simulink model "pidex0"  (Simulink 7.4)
settings: Solver=ode45  StartTime=0.0  StopTime=100  MaxStep=1e-3  RelTol=1e-3
libraries: simulink x2

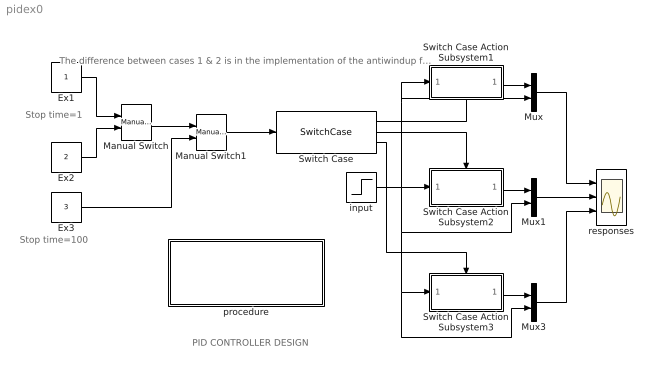
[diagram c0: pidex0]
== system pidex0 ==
  note: PID CONTROLLER DESIGN
  note: The difference between cases 1 & 2 is in the implementation of the antiwindup feature
  note: Stop time=1
  note: Stop time=100
  Ex1 : Constant  OutDataType=sfix(16)  OutScaling=2^0
  Ex2 : Constant  Value=2  OutDataType=sfix(16)  OutScaling=2^0
  Ex3 : Constant  Value=3  OutDataType=sfix(16)  OutScaling=2^0
  Manual Switch : simulink/Signal Routing/Manual Switch  SystemSampleTime=-1  sw=0  action=0  varsize=off
  Manual Switch1 : simulink/Signal Routing/Manual Switch  SystemSampleTime=-1  sw=0  action=0  varsize=off
  Mux : Mux  Inputs=2
  Mux1 : Mux  Inputs=2
  Mux3 : Mux  Inputs=2
  Switch Case : SwitchCase  CaseConditions={1,2,3}  ShowDefaultCase=off
  Switch Case Action Subsystem1 : Subsystem  TreatAsAtomicUnit=on
  Switch Case Action Subsystem2 : Subsystem  TreatAsAtomicUnit=on
  Switch Case Action Subsystem3 : Subsystem  TreatAsAtomicUnit=on
  input : Step  Time=.05  SampleTime=0
  procedure : Subsystem
  responses : Scope  NumInputPorts=3
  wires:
  Ex1/1 -> Manual Switch/1
  Ex2/1 -> Manual Switch/2
  Switch Case/2 -> Switch Case Action Subsystem2/Action
  Switch Case/1 -> Switch Case Action Subsystem1/Action
  input/1 -> Switch Case Action Subsystem2/1(In1), Mux1/2, Mux3/2, Switch Case Action Subsystem3/1(In1), Switch Case Action Subsystem1/1(In1), Mux/2
  Switch Case Action Subsystem1/1(Out1) -> Mux/1
  Switch Case Action Subsystem2/1(Out1) -> Mux1/1
  Mux1/1 -> responses/2
  Switch Case Action Subsystem3/1(Out1) -> Mux3/1
  Mux/1 -> responses/1
  Mux3/1 -> responses/3
  Switch Case/3 -> Switch Case Action Subsystem3/Action
  Manual Switch/1 -> Manual Switch1/1
  Manual Switch1/1 -> Switch Case/1
  Ex3/1 -> Manual Switch1/2

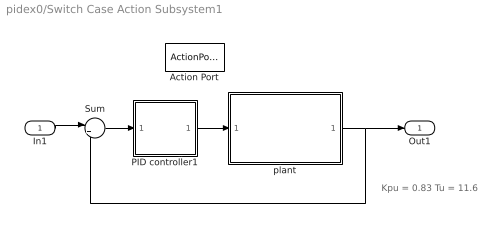
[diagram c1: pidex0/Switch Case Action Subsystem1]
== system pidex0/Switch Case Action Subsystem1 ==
  note: Kpu = 0.83 Tu = 11.6
  In1 : Inport  OutDataType=sfix(16)  OutScaling=2^0
  Action Port : ActionPort  ActionType=case
  PID controller1 : Subsystem  mask{Kp=5.1, Ki=53.7, Kd=0.11, sat=1.8}
      mask prompts: Kp "Proportional gain (Kp)"; Ki "Integral gain (Ki)"; Kd "Derivative gain (Kd)"; sat "Saturation limit [pu]"
      mask help: Proportional-Integral Speed Controller
  Sum : Sum  Inputs=|+-  OutDataType=sfix(16)  OutScaling=2^0
  plant : Subsystem  mask{Ka=1, Ta=0.25, Td=0.05}
      mask prompts: Ka "Gain"; Ta "Time constant [s]"; Td "Time delay [s]"
  Out1 : Outport
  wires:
  In1/1 -> Sum/1
  PID controller1/1(c) -> plant/1(In1)
  Sum/1 -> PID controller1/1(er)
  plant/1(Out1) -> Out1/1, Sum/2

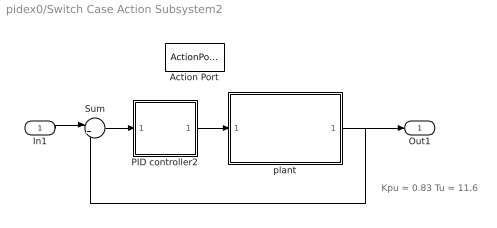
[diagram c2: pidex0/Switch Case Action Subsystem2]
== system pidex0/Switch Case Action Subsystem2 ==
  note: Kpu = 0.83 Tu = 11.6
  In1 : Inport  OutDataType=sfix(16)  OutScaling=2^0
  Action Port : ActionPort  ActionType=case
  PID controller2 : Subsystem  mask{Kp=5.1, Ki=53.7, Kd=0.11, sat=1.8}
      mask prompts: Kp "Proportional gain (Kp)"; Ki "Integral gain (Ki)"; Kd "Derivative gain (Kd)"; sat "Saturation limit [pu]"
      mask help: Proportional-Integral Speed Controller
  Sum : Sum  Inputs=|+-  OutDataType=sfix(16)  OutScaling=2^0
  plant : Subsystem  mask{Ka=1, Ta=0.25, Td=0.05}
      mask prompts: Ka "Gain"; Ta "Time constant [s]"; Td "Time delay [s]"
  Out1 : Outport
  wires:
  PID controller2/1(c) -> plant/1(In1)
  Sum/1 -> PID controller2/1(er)
  plant/1(Out1) -> Out1/1, Sum/2
  In1/1 -> Sum/1

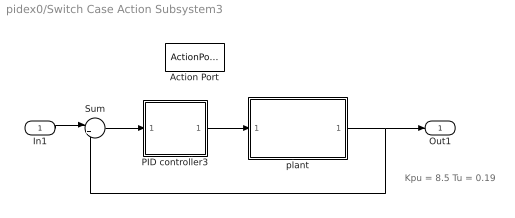
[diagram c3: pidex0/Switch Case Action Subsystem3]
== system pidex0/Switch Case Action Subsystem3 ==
  note: Kpu = 8.5 Tu = 0.19
  In1 : Inport  OutDataType=sfix(16)  OutScaling=2^0
  Action Port : ActionPort  ActionType=case
  PID controller3 : Subsystem  mask{Kp=0.5, Ki=0.09, Kd=0.77, sat=inf}
      mask prompts: Kp "Proportional gain (Kp)"; Ki "Integral gain (Ki)"; Kd "Derivative gain (Kd)"; sat "Saturation limit [pu]"
      mask help: Proportional-Integral Speed Controller
  Sum : Sum  Inputs=|+-  OutDataType=sfix(16)  OutScaling=2^0
  plant : Subsystem
  Out1 : Outport
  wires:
  In1/1 -> Sum/1
  PID controller3/1(c) -> plant/1(In1)
  Sum/1 -> PID controller3/1(er)
  plant/1(Out1) -> Out1/1, Sum/2

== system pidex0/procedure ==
  note: The controller parameters are obtained by first operating in a linear mode (setting sat=inf). In the presence of a limiter, an antiwindup action is often required as shown here in two different implementations of the antiwindup feature given in cases 1 and 2.
  note: P controller: Kp = 0.5*Kpu Ki = 0 Kd = 0 PI controller : Kp = 0.45*Kpu Ki = 0.54*Kpu/Tu Kd = 0 PID controller: Kp = 0.6*Kpu Ki = 1.2*Kpu/Tu Kd = 0.075*Kpu*Tu
  note: PID parameter tuning
  note: The transfer function of a PID controller is often written in this form: Gpid(s) = Kp + Ki/s + Kd*s Step 1: Set Ki = 0 and Kd = 0. Increase Kp in steps until the closed-loop response reaches a state of sustained oscillations. Mark this so-called ultimate gain denoted as Kpu. Measure the corresponding period of oscillation at the output , call it Tu. Step 2: Now set the parameters of the controller in accordance with the Ziegler-Nichols tuning criterion.

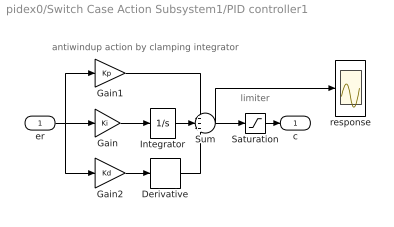
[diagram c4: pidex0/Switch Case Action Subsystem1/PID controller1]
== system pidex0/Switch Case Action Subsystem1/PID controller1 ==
  note: limiter
  note: antiwindup action by clamping integrator
  er : Inport  OutDataType=sfix(16)  OutScaling=2^0
  Derivative : Derivative
  Gain : Gain  Gain=Ki  ParameterDataType=sfix(16)  ParameterScaling=2^0  OutDataType=sfix(16)  OutScaling=2^0
  Gain1 : Gain  Gain=Kp  ParameterDataType=sfix(16)  ParameterScaling=2^0  OutDataType=sfix(16)  OutScaling=2^0
  Gain2 : Gain  Gain=Kd  ParameterDataType=sfix(16)  ParameterScaling=2^0  OutDataType=sfix(16)  OutScaling=2^0
  Integrator : Integrator  LimitOutput=on  UpperSaturationLimit=sat  LowerSaturationLimit=-sat
  Saturation : Saturate  UpperLimit=sat  LowerLimit=-sat
  Sum : Sum  Inputs=+++  OutDataType=sfix(16)  OutScaling=2^0
  response : Scope
  c : Outport  InitialOutput=0
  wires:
  Derivative/1 -> Sum/3
  Gain2/1 -> Derivative/1
  Integrator/1 -> Sum/2
  Saturation/1 -> c/1
  Sum/1 -> Saturation/1, response/1
  er/1 -> Gain2/1, Gain1/1, Gain/1
  Gain/1 -> Integrator/1
  Gain1/1 -> Sum/1

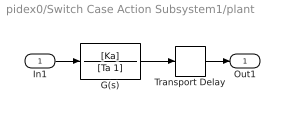
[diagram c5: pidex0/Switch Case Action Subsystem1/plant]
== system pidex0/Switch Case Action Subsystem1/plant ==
  In1 : Inport  OutDataType=sfix(16)  OutScaling=2^0
  G(s) : TransferFcn  Numerator=[Ka]  Denominator=[Ta 1]
  Transport Delay : TransportDelay  DelayTime=Td  BufferSize=2048
  Out1 : Outport
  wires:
  Transport Delay/1 -> Out1/1
  In1/1 -> G(s)/1
  G(s)/1 -> Transport Delay/1

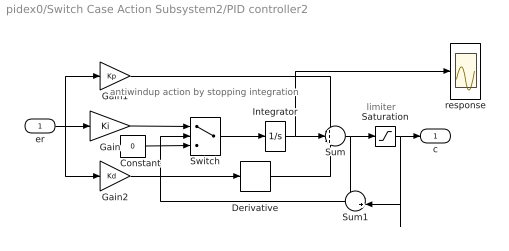
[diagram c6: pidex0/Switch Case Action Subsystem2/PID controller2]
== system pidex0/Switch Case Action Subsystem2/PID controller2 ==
  note: limiter
  note: antiwindup action by stopping integration
  er : Inport  OutDataType=sfix(16)  OutScaling=2^0
  Constant : Constant  Value=0  OutDataType=sfix(16)  OutScaling=2^0
  Derivative : Derivative
  Gain : Gain  Gain=Ki  ParameterDataType=sfix(16)  ParameterScaling=2^0  OutDataType=sfix(16)  OutScaling=2^0
  Gain1 : Gain  Gain=Kp  ParameterDataType=sfix(16)  ParameterScaling=2^0  OutDataType=sfix(16)  OutScaling=2^0
  Gain2 : Gain  Gain=Kd  ParameterDataType=sfix(16)  ParameterScaling=2^0  OutDataType=sfix(16)  OutScaling=2^0
  Integrator : Integrator
  Saturation : Saturate  UpperLimit=sat  LowerLimit=-sat
  Sum : Sum  Inputs=+++  OutDataType=sfix(16)  OutScaling=2^0
  Sum1 : Sum  Inputs=-+  OutDataType=sfix(16)  OutScaling=2^0
  Switch : Switch
  response : Scope
  c : Outport  InitialOutput=0
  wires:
  Switch/1 -> Integrator/1
  Sum1/1 -> Switch/2
  Constant/1 -> Switch/3
  Integrator/1 -> Sum/2, response/1
  Gain/1 -> Switch/1
  Saturation/1 -> Sum1/2, c/1
  Sum/1 -> Sum1/1, Saturation/1
  Gain2/1 -> Derivative/1
  Derivative/1 -> Sum/3
  er/1 -> Gain/1, Gain2/1, Gain1/1
  Gain1/1 -> Sum/1

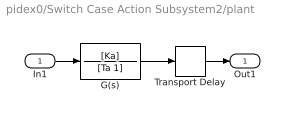
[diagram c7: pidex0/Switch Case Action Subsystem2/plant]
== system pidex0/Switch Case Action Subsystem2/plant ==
  In1 : Inport  OutDataType=sfix(16)  OutScaling=2^0
  G(s) : TransferFcn  Numerator=[Ka]  Denominator=[Ta 1]
  Transport Delay : TransportDelay  DelayTime=Td  BufferSize=2048
  Out1 : Outport
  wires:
  Transport Delay/1 -> Out1/1
  In1/1 -> G(s)/1
  G(s)/1 -> Transport Delay/1

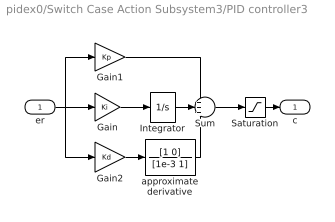
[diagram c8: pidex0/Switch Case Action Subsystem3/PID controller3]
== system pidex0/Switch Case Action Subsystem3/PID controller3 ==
  er : Inport  OutDataType=sfix(16)  OutScaling=2^0
  Gain : Gain  Gain=Ki  ParameterDataType=sfix(16)  ParameterScaling=2^0  OutDataType=sfix(16)  OutScaling=2^0
  Gain1 : Gain  Gain=Kp  ParameterDataType=sfix(16)  ParameterScaling=2^0  OutDataType=sfix(16)  OutScaling=2^0
  Gain2 : Gain  Gain=Kd  ParameterDataType=sfix(16)  ParameterScaling=2^0  OutDataType=sfix(16)  OutScaling=2^0
  Integrator : Integrator  LimitOutput=on  UpperSaturationLimit=sat  LowerSaturationLimit=-sat
  Saturation : Saturate  UpperLimit=sat  LowerLimit=-sat
  Sum : Sum  Inputs=+++  OutDataType=sfix(16)  OutScaling=2^0
  approximate derivative : TransferFcn  Numerator=[1 0]  Denominator=[1e-3 1]
  c : Outport  InitialOutput=0
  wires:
  Gain1/1 -> Sum/1
  Gain/1 -> Integrator/1
  er/1 -> Gain/1, Gain1/1, Gain2/1
  Sum/1 -> Saturation/1
  Saturation/1 -> c/1
  Integrator/1 -> Sum/2
  Gain2/1 -> approximate derivative/1
  approximate derivative/1 -> Sum/3

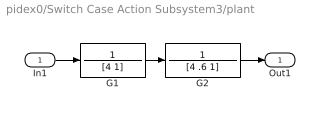
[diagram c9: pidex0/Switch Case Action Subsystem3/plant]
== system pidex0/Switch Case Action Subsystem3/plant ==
  In1 : Inport  OutDataType=sfix(16)  OutScaling=2^0
  G1 : TransferFcn  Numerator=1  Denominator=[4 1]
  G2 : TransferFcn  Numerator=1  Denominator=[4 .6 1]
  Out1 : Outport
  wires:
  G1/1 -> G2/1
  In1/1 -> G1/1
  G2/1 -> Out1/1
